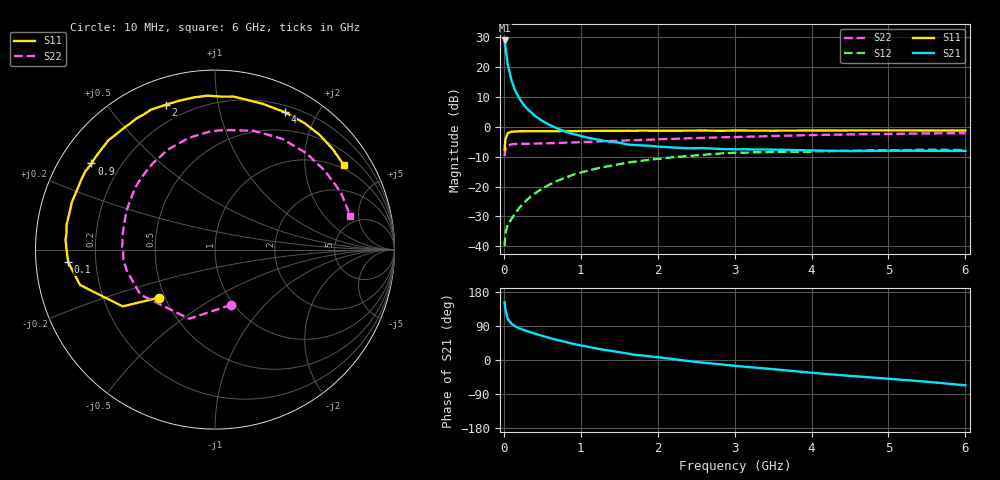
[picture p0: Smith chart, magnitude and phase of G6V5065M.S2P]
! SIEMENS Small Signal Semiconductors
! BFG193
! Si NPN RF Bipolar Junction Transistor in SOT223
! VCE = 0.5 V  IC = 65 mA
! Common Emitter S-Parameters:  August  1996
# GHz  S  MA  R  50
!  f  S11  S21  S12  S22
! GHz  MAG  ANG  MAG  ANG  MAG  ANG  MAG  ANG
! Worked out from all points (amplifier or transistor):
!   36 points, 10 MHz to 6 GHz, reference 50 ohm
!   highest |S21| = 28.7 dB at 10 MHz (marker M1)
!   |S21| within 3 dB of that: start of sweep to 24.19 MHz
!   unconditionally stable (mu >= 1): start of sweep to 17.84 MHz; 92.21 MHz to end of sweep
!   at 250 MHz: K = 1.33, MAG = 13.2 dB, |S12| = -25.7 dB
!   at 1.4 GHz: K = 1.29, MAG = 0.8 dB, |S12| = -13.0 dB
!   at 6 GHz: K = 1.07, MAG = -1.8 dB, |S12| = -7.8 dB
!   S11 on the Smith chart (normalised r, x): 10 MHz: 0.47, -0.30; 100 MHz: 0.10, -0.04; 900 MHz: 0.10, +0.31; 2 GHz: 0.12, +0.71; 4 GHz: 0.27, +1.60; 6 GHz: 0.87, +3.11
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0.01  0.4088 -139.2  27.37 152.1  0.0101 58.9  0.3209 -73.4
0.02  0.6037 -148.4  21.21 133.4  0.0164 49.1  0.4113 -110.5
0.05  0.7772 -165.3  11.1 108.4  0.0231 40.0  0.4857 -148.9
0.1  0.8211 -175.1  5.847 95.5  0.0289 46.6  0.5051 -166.6
0.15  0.8277 179.6  3.927 88.5  0.0363 52.1  0.5136 -173.7
0.2  0.8345 176.3  2.98 83.7  0.0437 55.9  0.5116 -178.0
0.25  0.8329 173.3  2.386 79.8  0.0516 58.4  0.5171 178.3
0.3  0.8386 170.7  2.001 76.3  0.0603 59.7  0.5168 175.9
0.4  0.8362 165.7  1.526 69.7  0.0761 60.7  0.5217 170.8
0.5  0.8404 161.4  1.245 63.7  0.0927 59.8  0.5238 166.5
0.7  0.8402 152.8  0.927 52.4  0.1251 56.7  0.5328 159.1
0.9  0.8391 145.1  0.754 42.8  0.1567 52.0  0.5439 151.5
1.1  0.8446 138.1  0.649 34.6  0.1849 47.1  0.5557 144.9
1.7  0.8514 117.6  0.492 13.7  0.2596 30.9  0.5933 125.0
2  0.8525 108.8  0.464 7.4  0.2893 22.2  0.6147 115.8
2.2  0.8533 103.4  0.448 2.4  0.3076 16.7  0.6236 109.6
2.8  0.853 87.5  0.424 -11.0  0.3544 0.9  0.6603 91.7
3.5  0.8546 71.9  0.413 -24.2  0.376 -17.5  0.6962 72.0
4  0.8588 63.0  0.4 -33.7  0.3824 -26.7  0.7216 58.9
4.5  0.8634 54.7  0.39 -41.9  0.3963 -36.0  0.7402 46.6
5.5  0.8626 40.4  0.394 -57.4  0.4126 -56.5  0.7706 24.4
6  0.8584 33.4  0.393 -66.7  0.4056 -68.2  0.7759 14.1
